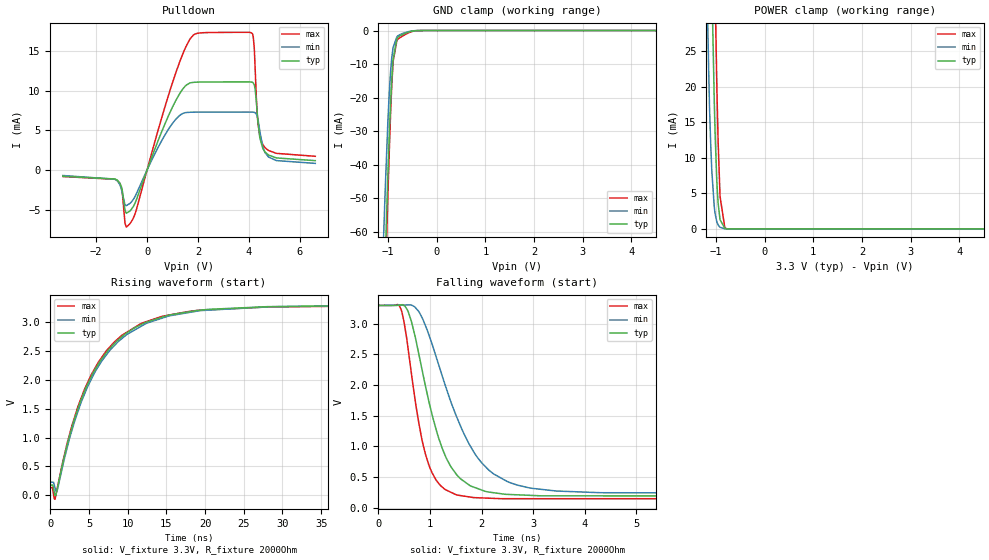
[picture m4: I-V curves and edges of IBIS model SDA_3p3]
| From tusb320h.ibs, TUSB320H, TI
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|   Model
[Model]   SDA_3p3
Model_type   I/O_open_drain
Polarity   Non-Inverting
Enable   Active-Low
Vinl = 0.99
Vinh = 2.31
Vmeas = 1.65
Vref = 3.3
Cref = 1pF
Rref = 2000
|   typ   min   max
C_comp   1pF   1pF   1pF
[Voltage Range]   3.3   3.299   3.301
[Temperature Range]   27   105   -40
[Pullup Reference]   3.3   3.299   3.301
[Pulldown Reference]   0   0   0
[Power Clamp Reference]   3.3   3.299   3.301
[GND Clamp Reference]   0   0   0
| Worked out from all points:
|   slope of the pulldown table from 0 to 0.495 V, typ, clamps not added: 118 ohm
|   GND clamp passes 1 mA (typ) near -0.67 V on its own axis
|   POWER clamp passes 1 mA (typ) near -0.89 V on its own axis
|   falling waveform, V_fixture 3.3V, R_fixture 2000Ohm: 20-80 % time 576ps typ, 865ps min, 386ps max; typ from 3.3 V to 0.179 V
|   rising waveform, V_fixture 3.3V, R_fixture 2000Ohm: 20-80 % time 6.6ns typ, 6.79ns min, 6.46ns max; typ from 0.179 V to 3.3 V
[Pulldown]
|   Voltage   I(typ)   I(min)   I(max)
-3.3V     -775.9uA   -683.3uA   -813uA
-1.152V   -1.313mA   -1.399mA   -1.356mA
-973.5mV  -2.521mA   -2.878mA   -2.699mA
-864.6mV  -5.035mA   -4.366mA   -6.666mA
-676.5mV  -5.168mA   -4.213mA   -6.781mA
1.264V    9.53mA     6.831mA    13.46mA
2.095V    11.08mA    7.296mA    17.27mA
4.125V    11.06mA    7.298mA    17.21mA
4.204V    10.73mA    7.263mA    15.44mA
4.353V    6.01mA     6.378mA    5.868mA
4.541V    2.737mA    2.92mA     3.21mA
6.6V      1.186mA    843.5uA    1.733mA
[GND Clamp]
|   Voltage   I(typ)   I(min)   I(max)
-3.3V     -1.349A    -1.276A    -1.4A
-1.112V   -95.92mA   -71.79mA   -106.5mA
-1.082V   -81.03mA   -58.65mA   -90.53mA
-1.053V   -66.59mA   -46.23mA   -74.95mA
-1.003V   -44mA      -27.89mA   -50.16mA
-973.5mV  -31.79mA   -18.89mA   -36.43mA
-924mV    -15.25mA   -8.461mA   -17.14mA
-894.3mV  -8.65mA    -5.039mA   -9.291mA
-815.1mV  -2.406mA   -1.841mA   -2.897mA
-726mV    -1.369mA   -1.037mA   -1.881mA
-369.6mV  -11.74uA   -10.2uA    -15.01uA
6.6V      0A         0A         0A
[POWER Clamp]
|   Voltage   I(typ)   I(min)   I(max)
-3.3V     1.3A       1.213A     1.36A
-1.221V   96.73mA    46.01mA    135.6mA
-1.132V   54.75mA    17.6mA     88.5mA
-1.082V   34.49mA    8.118mA    63.79mA
-1.013V   13mA       2.086mA    32.65mA
-983.4mV  7.256mA    1.097mA    21.47mA
-973.5mV  5.834mA    881.4uA    18.17mA
-953.7mV  3.655mA    566.6uA    12.4mA
-914.1mV  1.303mA    231.6uA    4.589mA
-815.1mV  79.27uA    24.14uA    151.9uA
-755.7mV  14.3uA     6.184uA    16.83uA
6.6V      0A         0A         0A
[Ramp]
R_load = 2000
|   typ   min   max
dV/dt_r   1.87248/6.60413e-09   1.84301/6.7851e-09   1.89986/6.453e-09
dV/dt_f   1.87248/5.75258e-10   1.84301/8.64854e-10   1.89986/3.83826e-10
[Falling Waveform]
V_fixture = 3.3V
V_fixture_min = 3.299V
V_fixture_max = 3.301V
R_fixture = 2000Ohm
C_fixture = 0F
|   Time   V(typ)   V(min)   V(max)
0s        3.3V       3.299V     3.301V
445ps     3.31V      3.306V     3.231V
643ps     3.039V     3.306V     2.191V
842.7ps   2.277V     3.11V      1.129V
1.115ns   1.295V     2.48V      457.8mV
1.406ns   669.4mV    1.729V     250.6mV
1.756ns   371mV      1.044V     174.8mV
2.388ns   224.9mV    477.6mV    144.8mV
4.354ns   191.1mV    242.2mV    144.7mV
200ns     179.2mV    227.3mV    134.6mV
[Rising Waveform]
V_fixture = 3.3V
V_fixture_min = 3.299V
V_fixture_max = 3.301V
R_fixture = 2000Ohm
C_fixture = 0F
|   Time   V(typ)   V(min)   V(max)
0s        179.2mV    227.3mV    134.6mV
594.6ps   6.248mV    137.6mV    -67.8mV
852.2ps   84.22mV    70.33mV    90.28mV
2.184ns   876.2mV    825.2mV    903.2mV
3.602ns   1.512V     1.461V     1.547V
7.195ns   2.457V     2.42V      2.491V
12.35ns   2.992V     2.971V     3.002V
17.93ns   3.175V     3.163V     3.182V
49.07ns   3.295V     3.293V     3.286V
200ns     3.3V       3.299V     3.301V
